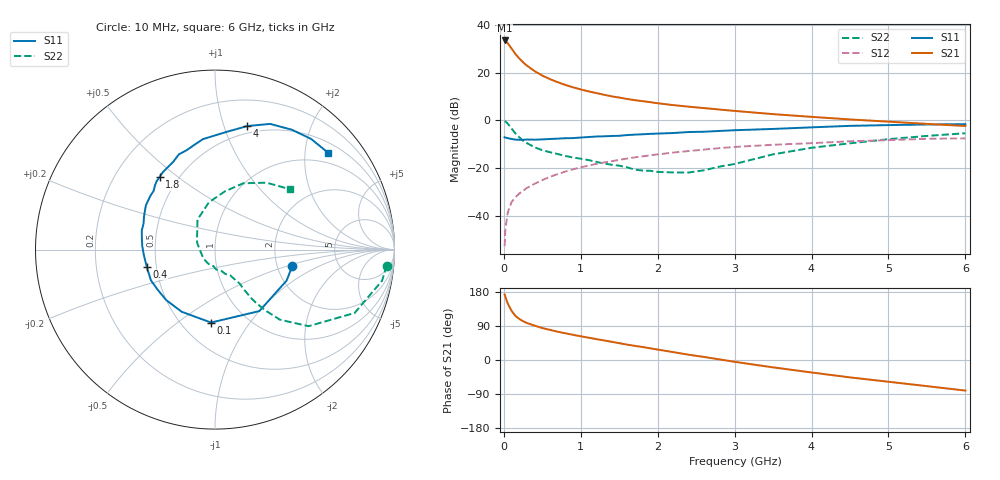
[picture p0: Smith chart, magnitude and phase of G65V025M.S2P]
! SIEMENS Small Signal Semiconductors
! BFG193
! Si NPN RF Bipolar Junction Transistor in SOT223
! VCE = 5 V  IC = 25 mA
! Common Emitter S-Parameters:  August  1996
# GHz  S  MA  R  50
!  f  S11  S21  S12  S22
! GHz  MAG  ANG  MAG  ANG  MAG  ANG  MAG  ANG
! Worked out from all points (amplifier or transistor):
!   36 points, 10 MHz to 6 GHz, reference 50 ohm
!   highest |S21| = 33.5 dB at 10 MHz (marker M1)
!   |S21| within 3 dB of that: start of sweep to 91.86 MHz
!   unconditionally stable (mu >= 1): 643.8 MHz to 2.38 GHz
!   at 250 MHz: K = 0.79, MSG = 26.9 dB, |S12| = -29.5 dB
!   at 1.4 GHz: K = 1.05, MAG = 12.3 dB, |S12| = -17.1 dB
!   at 6 GHz: K = 0.88, MSG = 2.6 dB, |S12| = -7.6 dB
!   S11 on the Smith chart (normalised r, x): 10 MHz: 2.43, -0.55; 100 MHz: 0.69, -0.67; 400 MHz: 0.44, -0.10; 1.8 GHz: 0.39, +0.43; 4 GHz: 0.43, +1.20; 6 GHz: 0.73, +2.51
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0.01  0.4404 -11.9  47.16 172.9  0.0023 90.6  0.9614 -5.3
0.02  0.4348 -23.4  46.05 167.0  0.0052 87.5  0.9465 -10.6
0.05  0.4224 -54.2  41.37 149.1  0.0115 72.4  0.8544 -24.4
0.1  0.4071 -93.1  32.03 129.9  0.0193 65.2  0.6737 -39.3
0.15  0.3929 -118.1  24.6 116.4  0.0244 60.8  0.5321 -47.2
0.2  0.3912 -134.1  19.86 108.6  0.0291 61.0  0.4419 -50.3
0.25  0.3901 -145.3  16.4 102.3  0.0334 61.1  0.374 -52.4
0.3  0.396 -154.4  14.01 97.7  0.0382 62.3  0.3329 -53.4
0.4  0.3923 -166.0  10.74 90.7  0.0469 62.9  0.2719 -54.0
0.5  0.3979 -176.0  8.646 84.3  0.0558 63.0  0.236 -54.0
0.6  0.4059 177.1  7.29 79.5  0.0654 62.9  0.2142 -55.0
0.7  0.4126 170.9  6.295 74.7  0.0746 62.1  0.1966 -56.7
0.9  0.4235 160.1  4.913 66.4  0.0939 59.6  0.1662 -59.4
1.1  0.4454 151.4  4.044 58.9  0.1122 57.0  0.1469 -67.0
1.4  0.4689 139.9  3.183 48.1  0.1389 51.3  0.1173 -79.2
1.8  0.5094 127.2  2.523 34.4  0.1751 43.4  0.0885 -102.8
2.2  0.5411 115.5  2.083 20.8  0.2103 34.5  0.0808 -142.6
3.5  0.6594 84.3  1.347 -19.4  0.3068 4.2  0.1935 120.3
4  0.7118 75.3  1.18 -32.9  0.3318 -5.5  0.2654 97.4
4.5  0.7647 66.3  1.042 -45.9  0.3635 -15.6  0.3295 80.3
5.5  0.8168 49.0  0.842 -69.0  0.4108 -39.0  0.4709 52.3
6  0.8292 40.7  0.759 -80.7  0.4179 -52.6  0.5353 39.0
